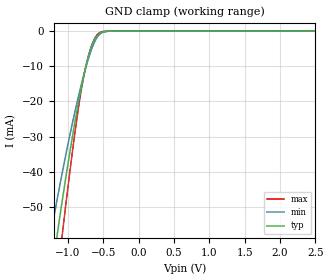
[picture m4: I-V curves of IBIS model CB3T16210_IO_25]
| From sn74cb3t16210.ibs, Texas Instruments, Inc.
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[Model]   CB3T16210_IO_25
Model_type  Terminator
| variable   typ   min   max
C_comp   3.80pF   3.13pF   4.48pF
| C_tri-state   3.80pF   3.13pF   4.48pF
[Temperature Range]   40   100   -40
| Ambient temperature   25   85   -40
[Voltage range]   2.5   2.3   2.7
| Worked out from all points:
|   GND clamp passes 1 mA (typ) near -0.57 V on its own axis
[GND Clamp]
| CB3T16210_IO_25
|   Voltage   I(typ)   I(min)   I(max)
-5.5V     -844.5mA   -703.3mA   -992.6mA
-1.255V   -72.43mA   -59.09mA   -89.08mA
-1.23V    -68.83mA   -56.29mA   -84.48mA
-1.14V    -56.21mA   -46.49mA   -68.25mA
-1.075V   -47.45mA   -39.7mA    -56.91mA
-910mV    -26.86mA   -23.7mA    -30.18mA
-790mV    -13.97mA   -13.54mA   -14.28mA
-730mV    -8.597mA   -9.13mA    -8.664mA
-670mV    -4.463mA   -5.382mA   -4.429mA
-560mV    -806.3uA   -1.072mA   -552.2uA
-340mV    -3.061uA   -5.509uA   -311.7nA
2.5V      185.2pA    1.95nA     72.59pA
